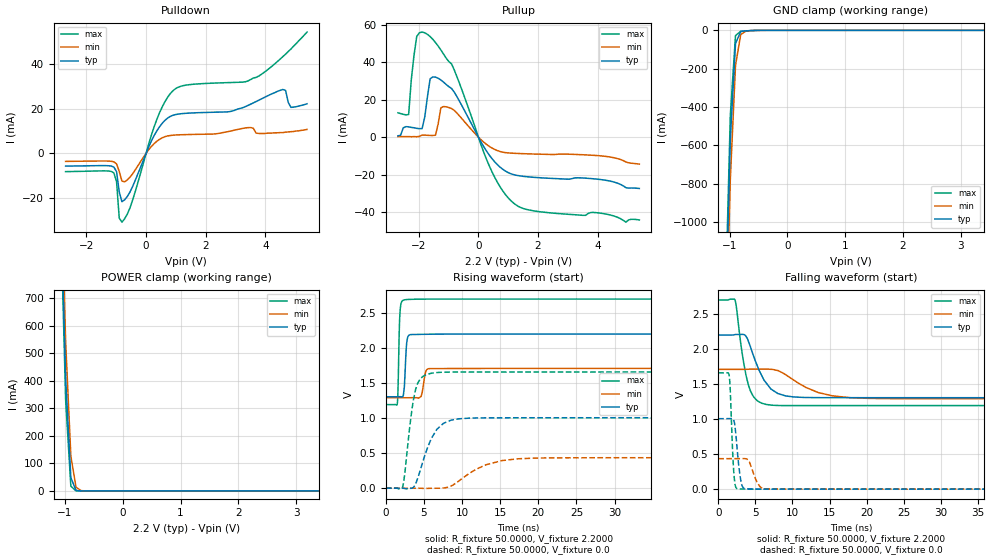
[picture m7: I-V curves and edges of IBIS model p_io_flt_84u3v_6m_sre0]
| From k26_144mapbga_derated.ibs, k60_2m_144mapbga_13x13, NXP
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[Model] p_io_flt_84u3v_6m_sre0
|   Model p_io_flt_84u3v_6m_sre0
| Library cells for typ/min/max conditions are connected as defined below:
|  pad - External Pad
|  ipp_do - Core Input
|  ipp_obe - Output Buffer Enable
|  esd_boost - vdd_s_3v
|  esd_bus - vdd_s_3v
|  ipp_do_3v - vss_bulk
|  ipp_ibe - vss_s_lv
|  ipp_ibe_3v - vss_bulk
|  ipp_ina40a_3v - NC
|  ipp_ina40b_3v - NC
|  ipp_ina_3v - NC
|  ipp_ind - NC
|  ipp_ind_3v - NC
|  ipp_obe1_3v - vss_bulk
|  ipp_pue - vss_s_lv
|  ipp_pue_3v - vss_bulk
|  ipp_pus - vss_s_lv
|  ipp_pus_3v - vss_bulk
|  ipp_sre - vss_s_lv
|  ipp_sre_3v - vss_bulk
|  ipt_mode_sw_3v - vss_bulk
|  vdd_s_3v - vdd_s_3v
|  vdd_s_lv - vdd_s_lv
|  vss_bulk - vss_bulk
|  vss_s_lv - vss_s_lv
| All other pins connected to ground
Model_type I/O
Polarity   Non-Inverting
Enable   Active-High
Vinl =   0.6600V
Vinh =   1.6500V
Vmeas =  1.1000V
Cref =   25.0000pF
Rref =   50.0000
Vref =   0.0V
C_comp   2.3415pF   2.1611pF   2.5701pF
[Temperature Range]   25.0000   0.1250k   -40.0000
[Voltage Range]   2.2000V   1.7100V   2.7000V
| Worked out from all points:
|   slope of the pulldown table from 0 to 0.33 V, typ, clamps not added: 35.3 ohm
|   slope of the pullup table from 0 to 0.33 V, typ, clamps not added: 37.5 ohm
|   GND clamp passes 1 mA (typ) near -0.60 V on its own axis
|   POWER clamp passes 1 mA (typ) near -0.77 V on its own axis
|   rising waveform, R_fixture 50.0000, V_fixture 2.2000: 20-80 % time 251ps typ, 359ps min, 190ps max; typ from 1.3 V to 2.2 V
|   rising waveform, R_fixture 50.0000, V_fixture 0.0: 20-80 % time 2.14ns typ, 4.23ns min, 1.13ns max; typ from 0 V to 1.01 V
|   falling waveform, R_fixture 50.0000, V_fixture 2.2000: 20-80 % time 2.33ns typ, 4.46ns min, 1.37ns max; typ from 2.2 V to 1.3 V
|   falling waveform, R_fixture 50.0000, V_fixture 0.0: 20-80 % time 572ps typ, 949ps min, 384ps max; typ from 1.01 V to 0 V
[Pulldown]
|Voltage   I(typ)   I(min)   I(max)
-2.7V     -5.71mA    -3.6mA     -8.18mA
-1.08V    -6.144mA   -3.805mA   -8.764mA
-990mV    -8.209mA   -4.705mA   -12.65mA
-900mV    -17.31mA   -8.075mA   -28.99mA
-810mV    -21.63mA   -12.4mA    -30.82mA
-540mV    -17.33mA   -10.67mA   -24.42mA
360mV     10.04mA    5.404mA    15.16mA
900mV     17.03mA    8.127mA    28.01mA
3.69V     23.2mA     9.1mA      34.01mA
4.59V     28.6mA     9.3mA      43.32mA
4.86V     20.6mA     9.7mA      46.7mA
5.4V      22.2mA     10.7mA     54.3mA
[Pullup]
|Voltage   I(typ)   I(min)   I(max)
-2.7V     700uA      300uA      13mA
-2.34V    5.5mA      300uA      12.1mA
-2.25V    5.2mA      200uA      31mA
-2.07V    4.7mA      200uA      53.8mA
-1.8V     10.71mA    1.07mA     55.8mA
-1.62V    31.18mA    910uA      53.76mA
-1.44V    32.09mA    1.04mA     50.59mA
-1.26V    30.56mA    15.7mA     46.62mA
-810mV    24.05mA    14.29mA    35.92mA
450mV     -11.38mA   -5.776mA   -18.35mA
1.17V     -20.01mA   -8.612mA   -35.13mA
5.4V      -27.45mA   -14.41mA   -44.3mA
[GND_clamp]
|Voltage   I(typ)   I(min)   I(max)
-2.7V     -26.42A    -26.26A    -26.57A
-1.08V    -1.572A    -1.753A    -1.479A
-990mV    -567.4mA   -776.5mA   -443.7mA
-900mV    -68.84mA   -182.9mA   -27.16mA
-810mV    -6.423mA   -22.29mA   -5.195mA
-720mV    -2.652mA   -3.693mA   -3.053mA
-450mV    -86.97uA   -164.9uA   -52.14uA
5.4V      0A         0A         0A
[POWER_clamp]
|Voltage   I(typ)   I(min)   I(max)
-2.7V     17.33A     17.21A     17.45A
-1.08V    1.086A     1.196A     1.032A
-990mV    408mA      540.5mA    329.6mA
-900mV    48.33mA    126.8mA    17.23mA
-810mV    1.793mA    13.06mA    218.7uA
-720mV    55.06uA    999.7uA    2.492uA
-630mV    1.661uA    73.44uA    28.49nA
5.4V      0A         0A         0A
[Ramp]
| variable   typ   min   max
dV/dt_r  0.6033/2.1368n   0.2609/4.2301n   0.9953/1.1345n
dV/dt_f  0.5369/2.3273n   0.2514/4.4556n   0.9041/1.3732n
R_load = 50.0000
[Rising Waveform]
R_fixture= 50.0000
V_fixture= 2.2000
V_fixture_min= 1.7100
V_fixture_max= 2.7000
|time   V(typ)   V(min)   V(max)
0s        1.305V     1.291V     1.193V
1.495ns   1.305V     1.291V     1.2V
1.596ns   1.305V     1.291V     1.421V
1.864ns   1.306V     1.291V     2.524V
2.421ns   1.442V     1.291V     2.688V
2.735ns   2.076V     1.291V     2.693V
3.238ns   2.192V     1.291V     2.696V
4.623ns   2.196V     1.31V      2.699V
5.661ns   2.198V     1.706V     2.699V
50ns      2.2V       1.71V      2.7V
[Rising Waveform]
R_fixture= 50.0000
V_fixture= 0.0
V_fixture_min= 0.0
V_fixture_max= 0.0
|time   V(typ)   V(min)   V(max)
0s        1.247nV    38.99nV    73.88pV
2.172ns   -113.5uV   33.98nV    7.955mV
3.387ns   -1.685mV   -6.971uV   1.099V
3.894ns   61.45mV    -2.94uV    1.407V
5.383ns   554.9mV    -4.283mV   1.625V
6.688ns   839.9mV    -1.195mV   1.651V
9.518ns   989.5mV    97.88mV    1.658V
13.14ns   1.004V     334.4mV    1.658V
17.41ns   1.005V     419.8mV    1.659V
50ns      1.006V     434.8mV    1.659V
[Falling Waveform]
R_fixture= 50.0000
V_fixture= 2.2000
V_fixture_min= 1.7100
V_fixture_max= 2.7000
|time   V(typ)   V(min)   V(max)
0s        2.2V       1.71V      2.7V
2.259ns   2.206V     1.71V      2.702V
3.235ns   2.209V     1.71V      1.935V
4.048ns   2.117V     1.712V     1.495V
4.913ns   1.857V     1.714V     1.3V
6.172ns   1.557V     1.714V     1.218V
9.077ns   1.331V     1.635V     1.193V
13.48ns   1.306V     1.379V     1.194V
17.89ns   1.306V     1.305V     1.194V
50ns      1.305V     1.291V     1.193V
[Falling Waveform]
R_fixture= 50.0000
V_fixture= 0.0
V_fixture_min= 0.0
V_fixture_max= 0.0
|time   V(typ)   V(min)   V(max)
0s        1.006V     434.9mV    1.659V
1.494ns   1.006V     434.7mV    1.613V
1.616ns   1.006V     434.7mV    1.437V
1.904ns   1.009V     434.6mV    633.9mV
2.124ns   972.9mV    434.6mV    203.1mV
2.605ns   513.5mV    434.7mV    5.662mV
3.109ns   91.53mV    435.7mV    2.071mV
3.707ns   5.615mV    434.2mV    1.293mV
6.303ns   760.5uV    4.139mV    501.9uV
50ns      139.3uV    73.04uV    195.4uV
